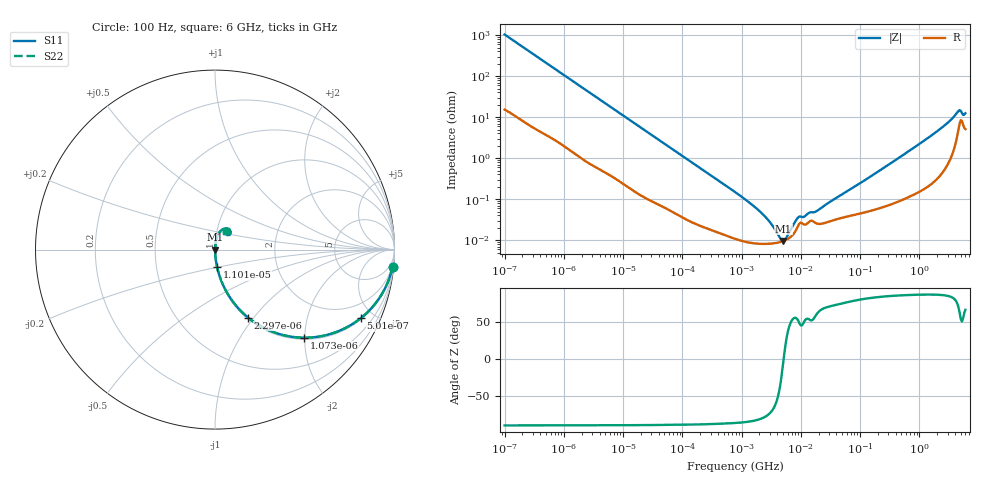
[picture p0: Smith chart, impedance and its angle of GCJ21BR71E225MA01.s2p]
!Murata Part Number: GCJ21BR71E225MA01
!These Parameters are Measured in Series Mode Connection
!Data Generated on Mar 13, 2026
!  o--ll--o
!Port1  Port2
!  o------o
!Operation Temp=25[degC], DC Bias Voltage=0[V]
!Freq. Start=100[Hz] Stop=6[GHz] 401[Steps]
# Hz S RI R 50
!Freq.(Hz) S11(Real) S11(Imag) S21(Real) S21(Imag) S12(Real) S12(Imag) S22(Real) S22(Imag)
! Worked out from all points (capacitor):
!   401 points, 100 Hz to 6 GHz, reference 50 ohm
!   read as one part in series: C = 1.52 uF near 109 Hz
!   lowest |Z| = 9.56 mohm at 5.079 MHz (marker M1)
!   series resonance near 5.136 MHz, so ESL is about 630 pH
!   S11 on the Smith chart (normalised r, x): 100 Hz: 1, -21; 501 Hz: 1.07, -4.22; 1.073 kHz: 1.04, -1.99; 2.297 kHz: 1.02, -0.94; 11.01 kHz: 1.00, -0.20; 6 GHz: 1.10, +0.23
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100  0.9895 -0.0949  0.0105 0.0949  0.0105 0.0949  0.9895 -0.0949
268  0.9358 -0.2374  0.0642 0.2374  0.0642 0.2374  0.9358 -0.2374
501  0.8125 -0.3817  0.1875 0.3817  0.1875 0.3817  0.8125 -0.3817
1073  0.498 -0.4908  0.502 0.4908  0.502 0.4908  0.498 -0.4908
2008  0.2272 -0.4101  0.7728 0.4101  0.7728 0.4101  0.2272 -0.4101
2297  0.1848 -0.3791  0.8152 0.3791  0.8152 0.3791  0.1848 -0.3791
4299  0.064 -0.235  0.936 0.235  0.936 0.235  0.064 -0.235
11009  0.012 -0.0984  0.988 0.0984  0.988 0.0984  0.012 -0.0984
40335  0.00149 -0.0276  0.9985 0.0276  0.9985 0.0276  0.00149 -0.0276
774597  0.00011 -0.00149  0.9999 0.00149  0.9999 0.00149  0.00011 -0.00149
2268635  8.12e-05 -0.000425  0.9999 0.000425  0.9999 0.000425  8.12e-05 -0.000425
3103719  8.23e-05 -0.000246  0.9999 0.000246  0.9999 0.000246  8.23e-05 -0.000246
4440638  8.97e-05 -6.93e-05  0.9999 6.93e-05  0.9999 6.93e-05  8.97e-05 -6.93e-05
5079039  9.54e-05 -5.3e-06  0.9999 5.3e-06  0.9999 5.3e-06  9.54e-05 -5.3e-06
5809218  0.000104 5.99e-05  0.9999 -5.99e-05  0.9999 -5.99e-05  0.000104 5.99e-05
9090158  0.000229 0.000281  0.9998 -0.000281  0.9998 -0.000281  0.000229 0.000281
1.555665e7  0.000296 0.000376  0.9997 -0.000376  0.9997 -0.000376  0.000296 0.000376
1.946e7  0.000251 0.000474  0.9997 -0.000474  0.9997 -0.000474  0.000251 0.000474
3.124326e8  0.000769 0.00711  0.9992 -0.00711  0.9992 -0.00711  0.000769 0.00711
1.95892e9  0.00495 0.0438  0.9951 -0.0438  0.9951 -0.0438  0.00495 0.0438
4.385646e9  0.0487 0.1157  0.9513 -0.1157  0.9513 -0.1157  0.0487 0.1157
6e9  0.0597 0.102  0.9403 -0.102  0.9403 -0.102  0.0597 0.102
